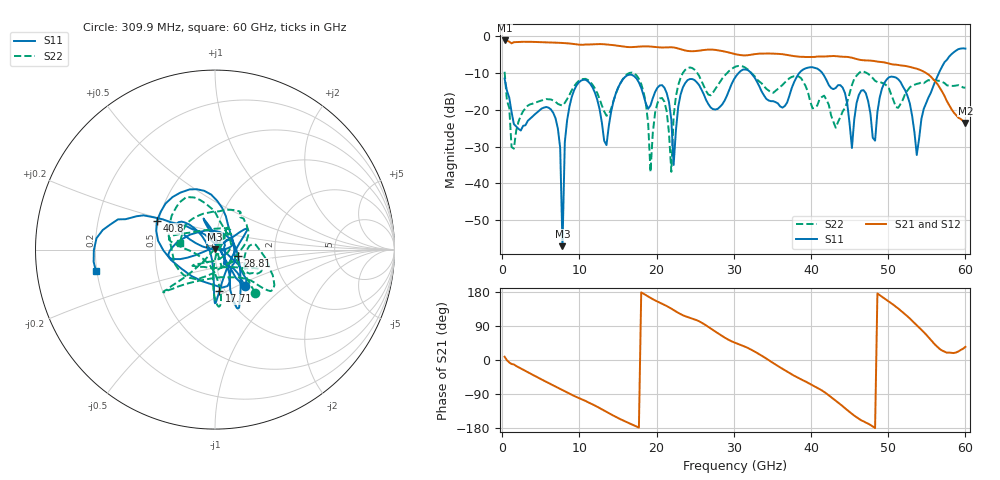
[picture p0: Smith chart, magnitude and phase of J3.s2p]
!Keysight Technologies,N5227A,US51270214,A.10.65.11
!Date: Thursday, October 15, 2020 08:18:16
!Correction: S11(Full 2 Port(1,2))
!S21(Full 2 Port(1,2))
!S12(Full 2 Port(1,2))
!S22(Full 2 Port(1,2))
!S2P File: Measurements: S11, S21, S12, S22:
# Hz S  dB  R 50
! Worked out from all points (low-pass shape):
!   200 points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, 309.9 MHz to 60 GHz, reference 50 ohm
!   highest |S21| = -1.22 dB at 309.9 MHz (marker M1); lowest = -23.6 dB at 60 GHz (marker M2)
!   |S21| within 3 dB of the highest: start of sweep to 28.8 GHz
!   lowest |S11| = -57.0 dB at 7.809 GHz (marker M3), VSWR 1.00, Z = 49.9 + j0.0573 ohm
!   |S11| at or under -10 dB: start of sweep to 30.64 GHz; 32.21 GHz to 38.51 GHz (6.302 GHz wide, 17.8 % of centre); 41.45 GHz to 56.58 GHz (15.14 GHz wide, 30.9 % of centre)
!   |S22| runs from -36.9 to -8.1 dB; largest |S21 - S12| = 0.13
!   S11 on the Smith chart (normalised r, x): 309.9 MHz: 1.27, -0.56; 17.71 GHz: 0.94, -0.46; 28.81 GHz: 1.29, -0.09; 40.8 GHz: 0.49, +0.18; 60 GHz: 0.20, -0.08
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3.0995e8  -11.56 -50.4  -1.22 8.6  -1.90 16.4  -9.71 -47.0
1.50975e9  -23.90 -29.6  -1.69 -11.8  -1.52 -10.6  -30.57 17.9
6.90885e9  -22.34 7.3  -1.82 -70.0  -1.80 -70.0  -17.87 70.3
7.50875e9  -30.31 -2.2  -1.86 -76.2  -1.85 -76.3  -18.68 90.5
7.8087e9  -57.02 156.0  -1.90 -79.4  -1.89 -79.4  -18.90 105.0
8.4086e9  -22.85 165.9  -1.98 -85.7  -1.99 -85.9  -17.13 132.6
1.050825e10  -11.89 145.2  -2.39 -105.3  -2.37 -105.6  -11.67 165.3
1.350775e10  -29.59 -137.5  -2.30 -136.8  -2.31 -136.8  -21.63 -138.5
1.770705e10  -12.62 -83.9  -2.87 -178.5  -2.89 -178.5  -11.64 -90.7
1.92068e10  -18.85 -1.8  -2.87 163.9  -2.89 163.9  -36.91 -40.4
2.04066e10  -13.42 31.7  -3.10 151.5  -3.12 151.5  -16.95 60.4
2.190635e10  -22.71 37.4  -3.06 135.5  -3.08 135.5  -36.85 -145.5
2.22063e10  -34.98 74.0  -3.11 131.8  -3.13 131.8  -21.73 -134.5
2.34061e10  -13.92 -164.7  -3.78 118.0  -3.80 118.1  -10.00 -140.1
2.88052e10  -17.54 -15.5  -4.22 59.3  -4.25 59.3  -10.77 -39.8
3.030495e10  -10.85 -60.6  -4.99 44.3  -5.00 44.3  -8.25 -36.7
4.02033e10  -8.48 137.0  -5.68 -66.7  -5.71 -66.9  -19.64 -73.2
4.08032e10  -8.85 153.8  -5.58 -73.3  -5.62 -73.3  -18.88 -122.0
4.530245e10  -30.38 35.9  -5.90 -142.1  -5.95 -142.0  -13.31 90.9
5.010165e10  -11.20 -53.3  -7.47 154.0  -7.49 154.4  -14.23 -121.4
5.370105e10  -32.28 39.9  -8.87 91.5  -8.91 91.7  -12.99 38.1
6e10  -3.42 -170.0  -23.63 34.8  -23.73 35.2  -14.04 169.4
